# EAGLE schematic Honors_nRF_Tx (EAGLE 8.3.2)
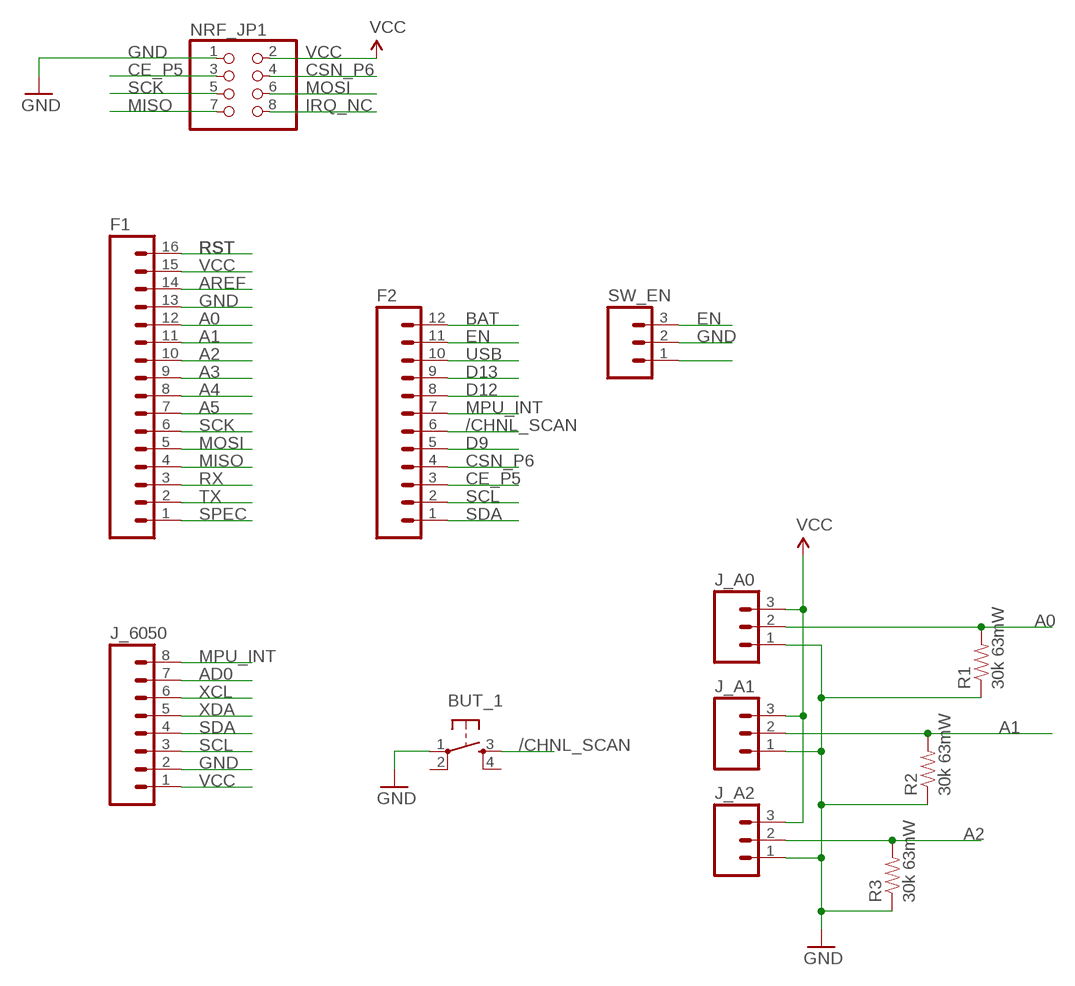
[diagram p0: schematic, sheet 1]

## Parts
BUT_1  TAC_SWITCHPTH  [TACTILE-PTH]
F1  M16PTH  [1X16]
F2  M12PTH  [1X12]
J_6050  M08  [1X08_ROUND]
J_A0  M03JST-PTH-VERT  [JST-3-PTH-VERT]
J_A1  M03JST-PTH-VERT  [JST-3-PTH-VERT]
J_A2  M03JST-PTH-VERT  [JST-3-PTH-VERT]
NRF_JP1  PINHD-2X4  [2X04]
R1  30k 63mW  RESISTOR1206  [1206]
R2  30k 63mW  RESISTOR1206  [1206]
R3  30k 63mW  RESISTOR1206  [1206]
SW_EN  M03PTH  [1X03]

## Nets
/CHNL_SCAN: BUT_1.3 F2.6
A0: F1.12 J_A0.2 R1.2
A1: F1.11 J_A1.2 R2.2
A2: F1.10 J_A2.2 R3.2
A3: F1.9
A4: F1.8
A5: F1.7
AD0: J_6050.7
AREF: F1.14
BAT: F2.12
CE_P5: F2.3 NRF_JP1.3
CSN_P6: F2.4 NRF_JP1.4
D9: F2.5
D12: F2.8
D13: F2.9
EN: F2.11 SW_EN.3
GND: BUT_1.1 F1.13 J_6050.2 J_A0.1 J_A1.1 J_A2.1 NRF_JP1.1 R1.1 R2.1 R3.1 SW_EN.2
IRQ_NC: NRF_JP1.8
MISO: F1.4 NRF_JP1.7
MOSI: F1.5 NRF_JP1.6
MPU_INT: F2.7 J_6050.8
N$3: SW_EN.1
RST: F1.16
RX: F1.3
SCK: F1.6 NRF_JP1.5
SCL: F2.2 J_6050.3
SDA: F2.1 J_6050.4
SPEC: F1.1
TX: F1.2
USB: F2.10
VCC: F1.15 J_6050.1 J_A0.3 J_A1.3 J_A2.3 NRF_JP1.2
XCL: J_6050.6
XDA: J_6050.5
Unconnected: BUT_1.2 BUT_1.4

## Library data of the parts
BUT_1 = SparkFun-Retired:TAC_SWITCH: Momentary Switch Button commonly used for reset or general input. Spark Fun Electronics SKU : COM-00097 SMT- SWCH-08247
F1 = SparkFun-Connectors:M16: 1x16 .1" header
F2 = SparkFun-Connectors:M12: Header 12 Standard 12-pin 0.1" header. Use with straight break away headers (SKU : PRT-00116), right angle break away headers (PRT-00553), swiss pins (PRT-00743), machine pins (PRT-00117), and female headers (PRT-00115).
J_6050 = SparkFun-Connectors:M08: Header 8 Standard 8-pin 0.1" header. Use with straight break away headers (SKU : PRT-00116), right angle break away headers (PRT-00553), swiss pins (PRT-00743), machine pins (PRT-00117), and female headers (PRT-00115).; PROD_ID: CONN-08437
J_A0 J_A1 J_A2 SW_EN = SparkFun-Connectors:M03: Header 3 Standard 3-pin 0.1" header. Use with straight break away headers (SKU : PRT-00116), right angle break away headers (PRT-00553), swiss pins (PRT-00743), machine pins (PRT-00117), and female headers (PRT-00115). Molex polarized connector foot print use with SKU : PRT-08232 with associated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
NRF_JP1 = pinhead:PINHD-2X4: PIN HEADER
R1-R3 = SparkFun-Resistors:RESISTOR: Resistor

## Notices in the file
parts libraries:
SparkFun-Connectors: Licensing: Creative Commons ShareAlike 4.0 International - https://creativecommons.org/licenses/by-sa/4.0
